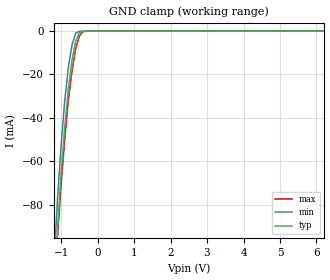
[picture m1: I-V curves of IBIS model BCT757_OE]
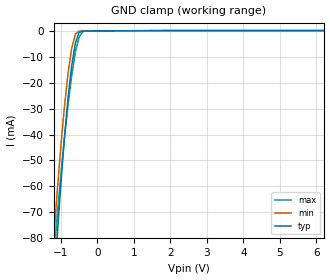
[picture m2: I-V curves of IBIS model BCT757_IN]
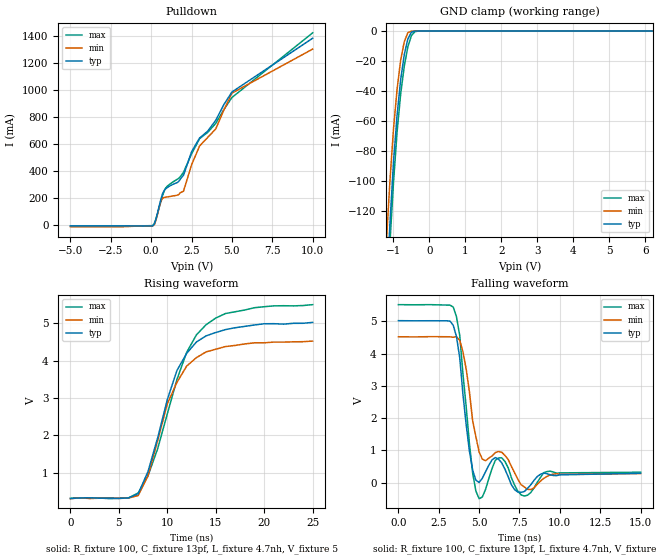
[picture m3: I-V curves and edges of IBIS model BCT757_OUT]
| TEXAS INSTRUMENTS INCORPORATED
| Standard Linear and Logic Group
| IBIS Model of SN64BCT757
| OCTAL BUFFER/DRIVER WITH OPEN-COLLECTOR OUTPUTS
| This file contains package information for the following:
|  SOIC 20-pin (DW) package as [Component] BCT757_DW
|  Plastic 20-pin (N) package as [Component] BCT757_N
| This device can be powered at the following Vccs:
|  5 volt Vcc
| This file provides unique models under the [Model Selector] for each Vcc.
| For operation at a specific Vcc, select the appropriate model after each
| [Model Selector] keyword.
[IBIS Ver]   3.2
[Comment char]  |_char
[File Name]   bct757.ibs
[File Rev]   1.1
[Date]   Feburary 11, 2004
[Source]   Data created from lab measurments at TI-SLL.
[Notes]   The following is an IBIS list for the BCT757.
   Please contact sllibis@ti.com with questions and
   comments concerning SLL IBIS models.
|   - All test data contained in this file are derived from
|   actual measurements.
|   - We have data across voltage and temperature, but not
|   across process.
|   - File created by Ernest Cox, SLL Applications.
[Disclaimer] Property of Texas Instruments Incorporated.  Unauthorized
   reproduction and/or distribution is strictly prohibited.
   This product is protected under copyright law.
   Created  2001, (C) Copyright  2001, Texas Instruments
   Incorporated, All Rights Reserved
   UNLESS THERE IS A SIGNED, WRITTEN AGREEMENT TO THE
   CONTRARY, TEXAS INSTRUMENTS (TI) IS PROVIDING THE IBIS
   MODELS  AND WITHOUT ANY WARRANTY, EXPRESSED OR
   IMPLIED.  TI assumes no liability for:
   1) the accuracy of the IBIS models provided to your
   company;
   2) the proper functioning of these IBIS Models in your
   design or for any resulting applications; or
   3) infringement of patents, copyrights or intellectual
   property rights resulting from your use of these IBIS
   models.
   TI provides IBIS Models as a service to our customers.
   You and your company shall not distribute, sell or give
   these models to anyone else without prior written
   permission from TI.
   TI reserves the right to make changes to our products or
   to discontinue any semiconductor product or service
   without notice, and advises our customers to obtain the
   latest version of relevant information to verify, before
   placing orders, that the information being relied on is
   current.
   Please be aware that your receipt and use of the IBIS
   information provided shall serve as acceptance of these
   terms and conditions.  If you do not accept these terms,
   you should return or destroy the IBIS models and any
   other accompanying information immediately.
| Component BCT757_DW 20-pin SOIC
[Component]   BCT757_DW
[Manufacturer]   Texas Instruments, Inc.
[Package]
|   typ   min   max
R_pkg   3.800e-02   3.300e-02   4.500e-02
L_pkg   5.012e-09   4.110e-09   6.349e-09
C_pkg   7.170e-13   5.300e-13   8.680e-13
[Pin]   signal_name   model_name   R_pin   L_pin   C_pin
1   1NOE   BCT757_OE   4.200e-02   6.336e-09   8.650e-13
2   1A1   BCT757_IN   4.300e-02   5.542e-09   8.670e-13
3   2Y4   BCT757_OUT   3.400e-02   4.714e-09   7.320e-13
4   1A2   BCT757_IN   3.400e-02   4.377e-09   5.910e-13
5   2Y3   BCT757_OUT   3.600e-02   4.130e-09   5.330e-13
6   1A3   BCT757_IN   3.500e-02   4.111e-09   5.300e-13
7   2Y2   BCT757_OUT   3.400e-02   4.284e-09   5.830e-13
8   1A4   BCT757_IN   3.400e-02   4.634e-09   7.260e-13
9   2Y1   BCT757_OUT   4.000e-02   5.518e-09   8.650e-13
10   GND   GND   4.300e-02   6.349e-09   8.660e-13
11   2A1   BCT757_IN   4.100e-02   6.281e-09   8.610e-13
12   1Y4   BCT757_OUT   4.500e-02   5.561e-09   8.680e-13
13   2A2   BCT757_IN   3.300e-02   4.778e-09   7.420e-13
14   1Y3   BCT757_OUT   3.500e-02   4.414e-09   5.960e-13
15   2A3   BCT757_IN   3.500e-02   4.110e-09   5.330e-13
16   1Y2   BCT757_OUT   3.600e-02   4.130e-09   5.330e-13
17   2A4   BCT757_IN   3.400e-02   4.377e-09   5.910e-13
18   1Y1   BCT757_OUT   3.400e-02   4.714e-09   7.310e-13
19   2OE   BCT757_OE   4.300e-02   5.569e-09   8.680e-13
20   VCC   POWER   4.200e-02   6.308e-09   8.640e-13
| Component BCT757_N 20-pin
[Component]   BCT757_N
[Manufacturer]   Texas   Instruments,   Inc.
[Package]
|   Mean.   Min.   Max.
R_pkg   0.043   0.038   0.05
L_pkg   7.384nH   4.68nH   10.321nH
C_pkg   0.51pF   0.231pF   0.821pF
[Pin]   signal_name   model_name   R_pin   L_pin   C_pin
1   1NOE   BCT757_OE   0.042   9.427nH   0.81pF
2   1A1   BCT757_IN   0.046   8.544nH   0.456pF
3   2Y4   BCT757_OUT   0.048   7.163nH   0.435pF
4   1A2   BCT757_IN   0.04   4.825nH   0.261pF
5   2Y3   BCT757_OUT   0.04   5.284nH   0.648pF
6   1A3   BCT757_IN   0.04   4.686nH   0.232pF
7   2Y2   BCT757_OUT   0.04   6.359nH   0.489pF
8   1A4   BCT757_IN   0.038   7.982nH   0.475pF
9   2Y1   BCT757_OUT   0.043   9.403nH   0.475pF
10   GND   GND   0.05   10.321nH   0.805pF
11   2A1   BCT757_IN   0.05   10.281nH   0.81pF
12   1Y4   BCT757_OUT   0.043   9.383nH   0.477pF
13   2A2   BCT757_IN   0.038   7.978nH   0.476pF
14   1Y3   BCT757_OUT   0.04   6.302nH   0.492pF
15   2A3   BCT757_IN   0.04   4.68nH   0.231pF
16   1Y2   BCT757_OUT   0.04   5.284nH   0.648pF
17   2A4   BCT757_IN   0.04   4.822nH   0.261pF
18   1Y1   BCT757_OUT   0.047   7.118nH   0.439pF
19   2OE   BCT757_OE   0.046   8.492nH   0.461pF
20   VCC   POWER   0.043   9.348nH   0.821pF
| Models and submodels in the file (3): BCT757_OE (Input), BCT757_IN (Input), BCT757_OUT (Open_drain)
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[Model]   BCT757_OE
Model_type  Input
Vinl=0.8
Vinh=2.0
| variable   typ   min   max
C_comp   5.4pF   4.9pF   5.9pF
[Temperature Range]   40   -40   100
| Ambient temperature   25   -40   85
[Voltage range]   5   4.5   5.5
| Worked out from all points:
|   GND clamp passes 1 mA (typ) near -0.51 V on its own axis
[GND Clamp]
| BCT757_OE
| Voltage   I(typ)   I(min)   I(max)
-5V       -1.42A     -1.55A     -1.3A
-1.2V     -122.6mA   -108.5mA   -123.8mA
-1.1V     -91.98mA   -77.52mA   -95.3mA
-1V       -65.62mA   -52.58mA   -70.53mA
-900mV    -44.39mA   -31.95mA   -49.87mA
-800mV    -26.44mA   -16.48mA   -31.51mA
-700mV    -13.44mA   -6.267mA   -18.22mA
-600mV    -4.718mA   -980.5uA   -8.186mA
-500mV    -681.2uA   -76.52uA   -2.235mA
-400mV    -69.74uA   -53.23uA   -253.6uA
-300mV    -42.47uA   -51.08uA   -55.51uA
10V       96.49pA    13.06nA    729.9pA
[Model]   BCT757_IN
Model_type  Input
Vinl=0.8
Vinh=2.0
| variable   typ   min   max
C_comp   5.9pF   5.6pF   6.1pF
[Temperature Range]   40   -40   85
| Ambient temperature   25   -40   70
[Voltage range]   5   4.5   5.5
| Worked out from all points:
|   GND clamp passes 1 mA (typ) near -0.51 V on its own axis
[GND Clamp]
| BCT757_IN
|Voltage   I(typ)   I(min)   I(max)
-5V       -1.3A      -1.1A      -887.8mA
-1.2V     -102.4mA   -81.46mA   -88.58mA
-1.1V     -79.45mA   -62.12mA   -71.6mA
-1V       -59.18mA   -44.61mA   -55.76mA
-900mV    -41.07mA   -29.13mA   -41.18mA
-800mV    -25.53mA   -16.06mA   -28.07mA
-700mV    -13.25mA   -6.677mA   -17mA
-600mV    -4.766mA   -1.308mA   -8.182mA
-500mV    -753.2uA   -186.3uA   -2.533mA
-400mV    -150.9uA   -150.4uA   -383.4uA
-300mV    -121.3uA   -144.8uA   -135.2uA
10V       15.32pA    10.09nA    929.1pA
[Model]   BCT757_OUT
Model_type  Open_drain
Enable   Active-Low
Vmeas =   2.5
| variable   typ   min   max
C_comp   12pF   11.4pF   12.9pF
[Temperature Range]   40   -40   85
| Ambient temperature   25   -40   70
[Voltage range]   5   4.5   5.5
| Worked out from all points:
|   slope of the pulldown table from 0 to 0.75 V, typ, clamps not added: 3.02 ohm
|   GND clamp passes 1 mA (typ) near -0.51 V on its own axis
|   falling waveform, R_fixture 100, C_fixture 13pf, L_fixture 4.7nh, V_fixture 5: 20-80 % time 598ps typ, 783ps min, 560ps max; typ from 5.02 V to 0.291 V
|   rising waveform, R_fixture 100, C_fixture 13pf, L_fixture 4.7nh, V_fixture 5: 20-80 % time 3.5ns typ, 3.34ns min, 3.91ns max; typ from 0.312 V to 5.02 V
[GND Clamp]
| BCT757_OUT
|Voltag   I(typ)   I(min)   I(max)
-5V       -2.8A      -2.55A     -2.6A
-1.2V     -178.2mA   -142.6mA   -189.7mA
-1.1V     -129.3mA   -100.7mA   -142.1mA
-1V       -87.72mA   -65.58mA   -101.3mA
-900mV    -56.27mA   -38.96mA   -67.45mA
-800mV    -32.41mA   -19.36mA   -42.04mA
-700mV    -15.74mA   -7.128mA   -23.47mA
-600mV    -5.254mA   -1.106mA   -10.52mA
-500mV    -745.7uA   -43.93uA   -3mA
-400mV    -41.24uA   -731.9nA   -370uA
-300mV    -1.21uA    -115.3nA   -23uA
10V       1.494nA    131.6nA    38.76nA
[Pulldown]
| BCT757_OUT
|Voltage  I(typ)   I(min)   I(max)
-5V       -5.34mA    -11.9mA    -5.1mA
100mV     -3.849mA   -3.96mA    -2.5mA
300mV     45.37mA    38.97mA    48.76mA
600mV     190.8mA    176.2mA    175.4mA
800mV     256.3mA    204.2mA    250.8mA
1.7V      322.2mA    226.2mA    345.4mA
2V        368.3mA    250.3mA    390.1mA
2.5V      541.5mA    445.5mA    526.3mA
3V        643.8mA    585.2mA    639mA
4V        774.6mA    710.9mA    751.8mA
5V        983.2mA    975.1mA    942.5mA
10V       1.38A      1.3A       1.42A
[Ramp]
| BCT757_OUT
| variable   typ   min   max
dV/dt_r   2.78/3.35E-9   2.66/3.50E-9   3.16/3.88E-9
dV/dt_f   2.86/6.0E-10   2.80/8.5E-10   3.34/5.7E-10
R_load =100
[Falling Waveform]
| BCT757_OUT
R_fixture =   100
C_fixture =   13pf
L_fixture =   4.7nh
V_fixture =   5
V_fixture_min = 4.5
V_fixture_max = 5.5
| Time   V(typ)   V(min)   V(max)
0s        5.022V     4.523V     5.519V
3.4ns     4.879V     4.509V     5.442V
3.8ns     3.873V     4.409V     4.562V
4ns       2.735V     4.06V      3.362V
4.6ns     389.1mV    1.922V     298.8mV
5ns       6.562mV    953.1mV    -497.5mV
6.2ns     729.4mV    968.1mV    766.2mV
7.8ns     -275.6mV   -132.5mV   -413.4mV
9.2ns     276.9mV    190.6mV    344.1mV
15ns      290.9mV    280.6mV    322.8mV
[Rising Waveform]
| BCT757_OUT
R_fixture =   100
C_fixture =   13pf
L_fixture =   4.7nh
V_fixture =   5
V_fixture_min = 4.5
V_fixture_max = 5.5
| Time   V(typ)   V(min)   V(max)
0s        312.2mV    304.7mV    310.3mV
7ns       440mV      390.3mV    459.4mV
8ns       1.027V     911.3mV    912.8mV
9ns       1.928V     1.854V     1.64V
10ns      2.957V     2.844V     2.575V
11ns      3.739V     3.421V     3.499V
12ns      4.193V     3.854V     4.223V
14ns      4.662V     4.233V     4.96V
19ns      4.953V     4.475V     5.415V
25ns      5.022V     4.522V     5.497V
